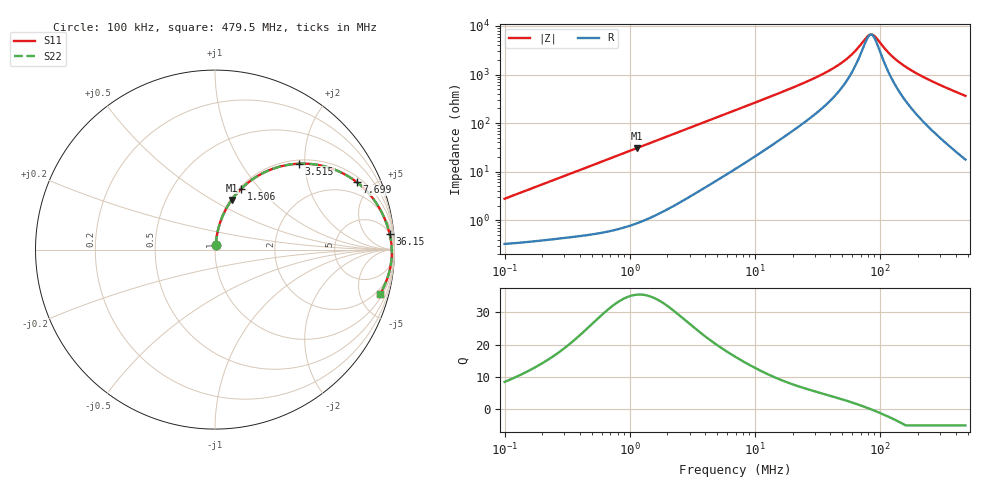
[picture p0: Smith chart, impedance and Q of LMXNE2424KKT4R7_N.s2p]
! LMXNE2424KKT4R7_N  S-PARAMETER MODEL  ( General Type )
! Model Generated by TAIYO YUDEN Corporation (http://www.ty-top.com)
! Version 1.0
! TAIYO YUDEN Control No. 191023NI43SB-FBB
! Copyright(c) 2019 TAIYO YUDEN CO.,LTD. All Rights Reserved.
! Product Description (link to TY-COMPAS)
! https://ds.yuden.co.jp/TYCOMPAS/or/detail?pn=LMXNE2424KKT4R7MN&u=M
! Products Name : Inductors
! Characteristics :
!  Inductance : 4.7 uH , SRF(min) : 50 MHz , DC Resistance(max) : 0.348 Ohm
!  Rated Current : Saturation :880 mA , Temp Rise : 670 mA
!  Case Size : 2.4 x 2.4 / 0.094 x 0.094 [mm/inch] , Thickness : 1 / 0.039 [mm/inch]
!  (Conditions: Temperature = 25 degC , DC Bias Current/Voltage = 0A / 0V)
! External Node Assignments :
!  1  o---GGG---o  2
! GND o---------o GND
! Frequency Range : 0.1MHz  -  479.524407MHz  [ 402 STEP ]
# MHz S RI R 50
! Freq[MHz].  S11 Real  S11 Imag  S21 Real  S21 Imag  S12 Real  S12 Imag  S22 Real  S22 Imag
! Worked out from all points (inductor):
!   401 points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, 100 kHz to 479.5 MHz, reference 50 ohm
!   read as one part in series: L = 4.36 uH near 104.3 kHz
!   highest Q = 35.4 at 1.143 MHz (marker M1), where L = 4.27 uH
!   self-resonance near 84.31 MHz
!   S11 on the Smith chart (normalised r, x): 100 kHz: 1.01, +0.05; 1.506 MHz: 1.02, +0.81; 3.515 MHz: 1.08, +1.87; 7.699 MHz: 1.27, +4.06; 36.15 MHz: 6, +21; 479.5 MHz: 1.36, -7.27
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0.1  0.00399 0.0273  0.996 -0.0273  0.996 -0.0273  0.00399 0.0273
0.413557  0.0169 0.1092  0.9831 -0.1092  0.9831 -0.1092  0.0169 0.1092
1.143492  0.0926 0.276  0.9074 -0.276  0.9074 -0.276  0.0926 0.276
1.506119  0.1472 0.3402  0.8528 -0.3402  0.8528 -0.3402  0.1472 0.3402
1.710297  0.1807 0.3702  0.8193 -0.3702  0.8193 -0.3702  0.1807 0.3702
3.515123  0.4682 0.4788  0.5318 -0.4788  0.5318 -0.4788  0.4682 0.4788
4.830264  0.6159 0.4623  0.3841 -0.4623  0.3841 -0.4623  0.6159 0.4623
7.073061  0.7638 0.3948  0.2362 -0.3948  0.2362 -0.3948  0.7638 0.3948
7.698666  0.7901 0.3757  0.2099 -0.3757  0.2099 -0.3757  0.7901 0.3757
13.64175  0.9083 0.2439  0.0917 -0.2439  0.0917 -0.2439  0.9083 0.2439
28.6379  0.9652 0.1161  0.0348 -0.1161  0.0348 -0.1161  0.9652 0.1161
36.15459  0.9731 0.0866  0.0269 -0.0866  0.0269 -0.0866  0.9731 0.0866
55.23368  0.9818 0.0409  0.0182 -0.0409  0.0182 -0.0409  0.9818 0.0409
64.06461  0.9835 0.0263  0.0165 -0.0263  0.0165 -0.0263  0.9835 0.0263
77.52404  0.9849 0.008  0.0151 -0.008  0.0151 -0.008  0.9849 0.008
82.61188  0.9852 0.00194  0.0148 -0.00194  0.0148 -0.00194  0.9852 0.00194
86.18795  0.9853 -0.00211  0.0147 0.00211  0.0147 0.00211  0.9853 -0.00211
91.84439  0.9854 -0.0082  0.0146 0.0082  0.0146 0.0082  0.9854 -0.0082
118.4342  0.985 -0.0333  0.015 0.0333  0.015 0.0333  0.985 -0.0333
149.52  0.983 -0.0581  0.017 0.0581  0.017 0.0581  0.983 -0.0581
201.1535  0.9776 -0.0942  0.0224 0.0942  0.0224 0.0942  0.9776 -0.0942
479.5244  0.9194 -0.2489  0.0806 0.2489  0.0806 0.2489  0.9194 -0.2489
